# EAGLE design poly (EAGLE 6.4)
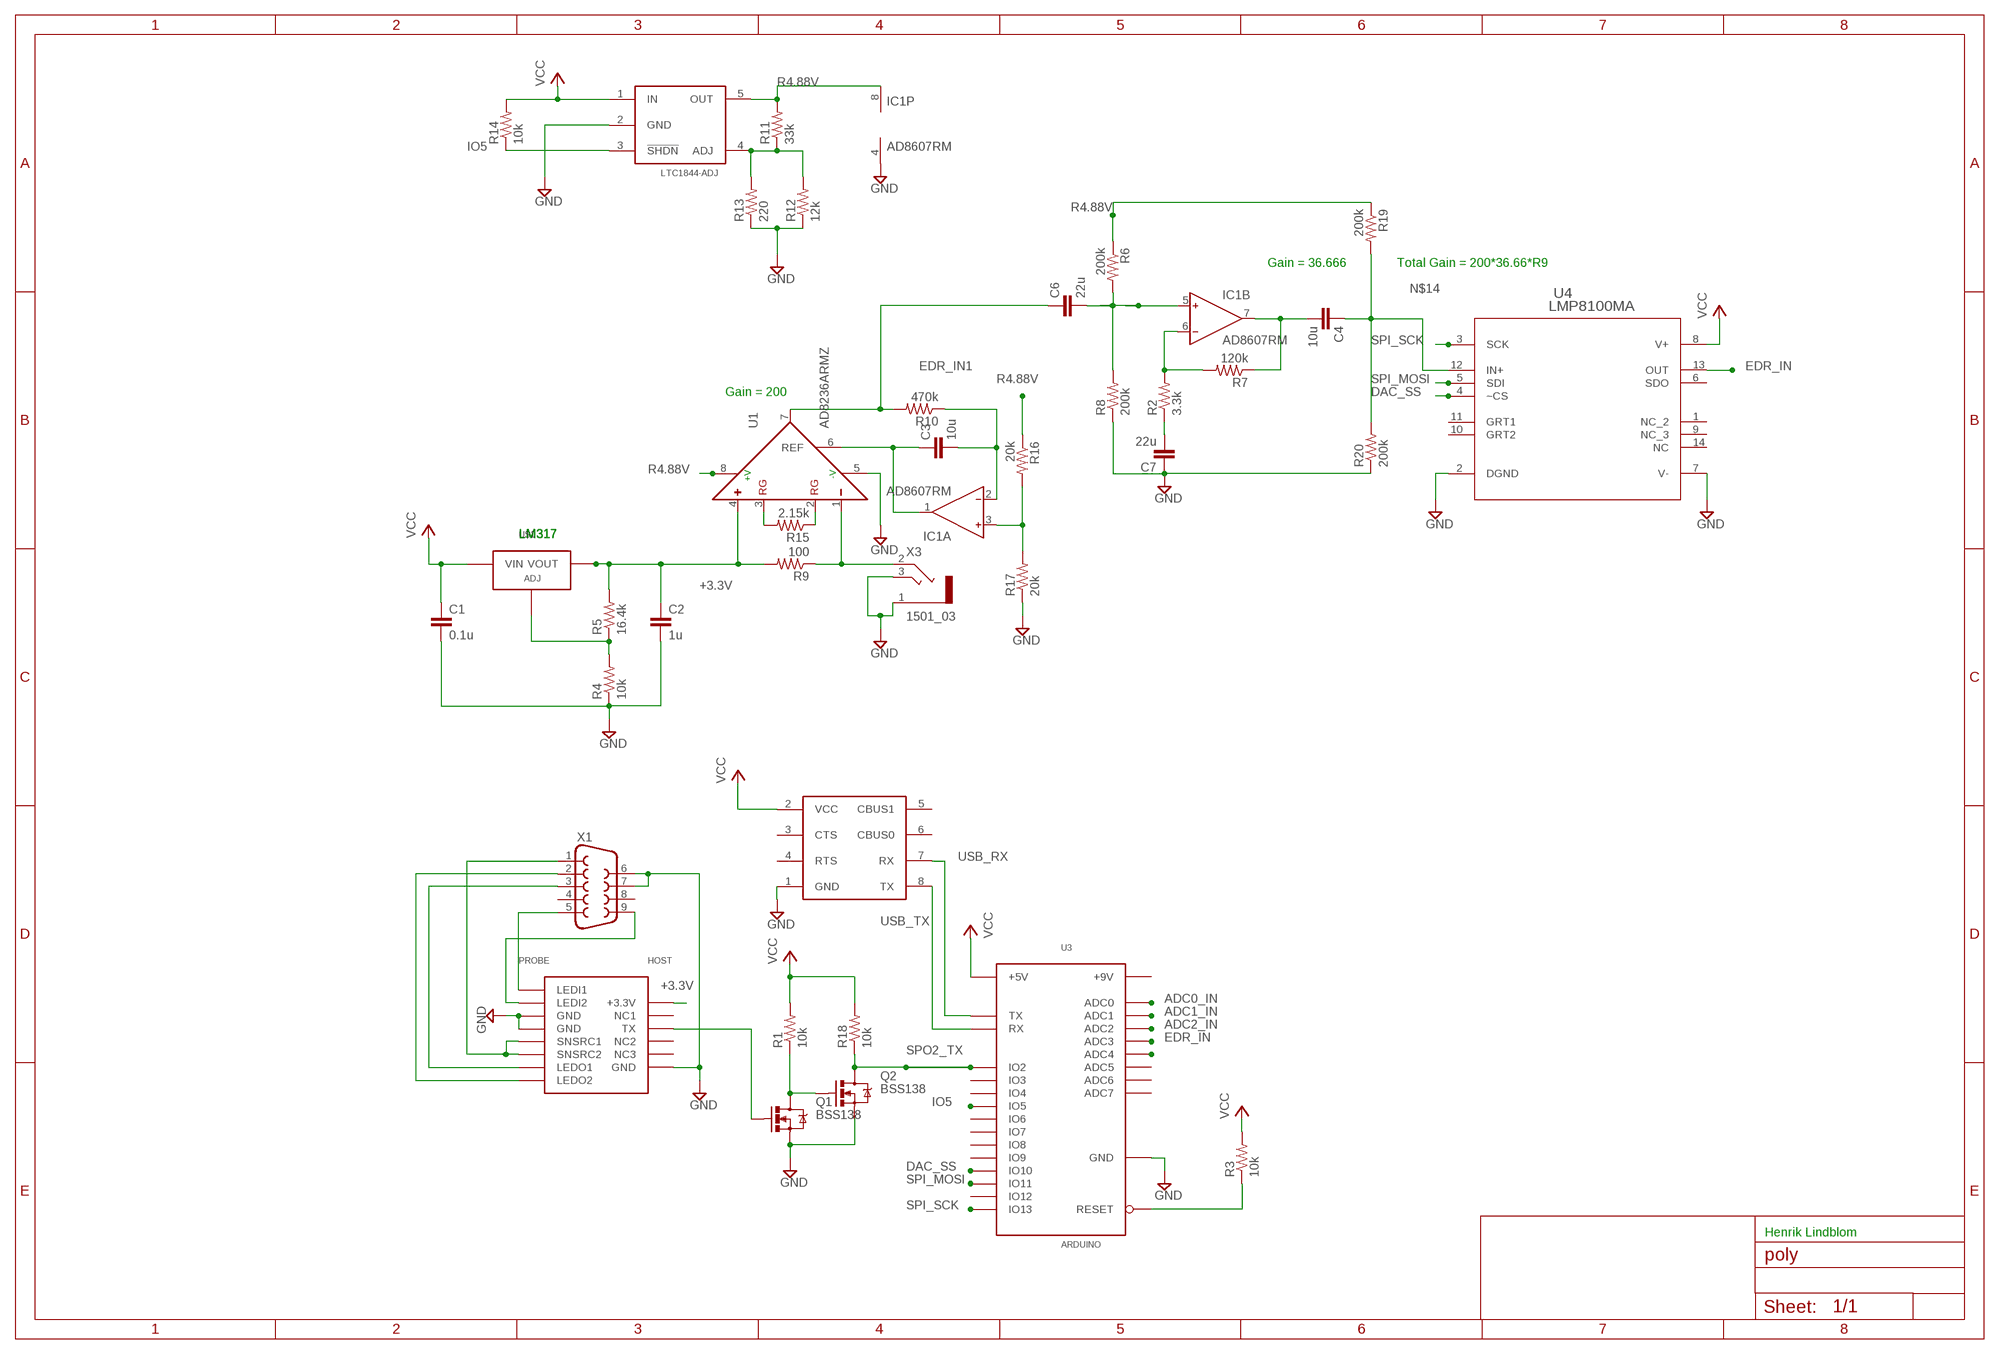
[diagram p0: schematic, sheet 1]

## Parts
C1  0.1u  C-EUC0603K  [C0603K]
C2  1u  C-EUC0805K  [C0805K]
C3  10u  C-EUC0805K  [C0805K]
C4  10u  C-EUC0603  [C0603]
C6  22u  C-EUC0805K  [C0805K]
C7  22u  C-EUC0805K  [C0805K]
IC1  AD8607RM  [MSOP08]
MEDLABSPO2  MEDLAB_SPO2  [MEDLAB_SPO2]
Q1  BSS138  BSS138TRANS-00830  [SOT23-3]
Q2  BSS138  BSS138TRANS-00830  [SOT23-3]
R1  10k  RESISTOR0805-RES  [0805]
R2  3.3k  RESISTOR0805-RES  [0805]
R3  10k  RESISTOR0805-RES  [0805]
R4  10k  RESISTOR0805-RES  [0805]
R5  16.4k  RESISTOR0805-RES  [0805]
R6  200k  RESISTOR0805-RES  [0805]
R7  120k  RESISTOR0805-RES  [0805]
R8  200k  RESISTOR0805-RES  [0805]
R9  100  RESISTOR0805-RES  [0805]
R10  470k  RESISTOR0805-RES  [0805]
R11  33k  RESISTOR0805-RES  [0805]
R12  12k  RESISTOR0805-RES  [0805]
R13  220  RESISTOR0805-RES  [0805]
R14  10k  RESISTOR0805-RES  [0805]
R15  2.15k  RESISTOR0805-RES  [0805]
R16  20k  RESISTOR0603-RES  [0603-RES]
R17  20k  RESISTOR0603-RES  [0603-RES]
R18  10k  RESISTOR0805-RES  [0805]
R19  200k  RESISTOR0603-RES  [0603-RES]
R20  200k  RESISTOR0603-RES  [0603-RES]
U1  AD8236ARMZ  [SOP65P490X110-8N]
U2  UB232R  [UB232R]
U3  ARDUINO  [ARDUINO_MINI]
U4  LMP8100MA  [M14A]
U$1  LM317  [SOT-89]
U$5  LTC1844-ADJ  [SOT23-5]
X1  F09HP  [F09HP]
X3  1501_03  [1501_03]

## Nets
+3.3V: C2.1 MEDLABSPO2.+3.3V R5.2 R9.2 U1.4(+) U$1.P$1(VOUT) U$1.P$2(VOUT)
ADC0_IN: U3.ADC0
ADC1_IN: U3.ADC1
ADC2_IN: U3.ADC2
ADC4_IN: U3.ADC4
DAC_SS: U3.IO10 U4.4(~CS)
EDR_IN: U3.ADC3 U4.13(OUT)
EDR_IN1: C3.2 IC1.2(A:IN-) R10.1
EDR_IN2: C4.2 IC1.7(B:OUT) R7.1
GND: C1.2 C2.2 C7.1 IC1.4(P:V-) MEDLABSPO2.GND MEDLABSPO2.GND@1(GND) MEDLABSPO2.GND@2(GND) Q1.2(S) Q2.2(S) R4.1 R8.1 R12.1 R13.1 R17.1 R20.1 U1.5(-V) U2.1(GND) U3.GND U4.2(DGND) U4.7(V-) U$5.2(GND) X1.6 X1.7 X3.1 X3.3
IO5: R14.1 U3.IO5 U$5.3(!SHDN)
N$1: MEDLABSPO2.LEDI1 X1.5
N$2: MEDLABSPO2.LEDI2 X1.9
N$3: MEDLABSPO2.SNSRC1 MEDLABSPO2.SNSRC2 X1.1
N$4: MEDLABSPO2.LEDO1 X1.3
N$5: MEDLABSPO2.LEDO2 X1.2
N$6: R3.1 U3.RESET
N$9: MEDLABSPO2.TX Q1.1(G)
N$10: Q1.3(D) Q2.1(G) R1.1
N$11: R4.2 R5.1 U$1.P$3(ADJ)
N$12: IC1.6(B:IN-) R2.2 R7.2
N$13: C6.1 R10.2 U1.7(OUT)
N$14: C4.1 R19.2 R20.2 U4.12(IN+)
N$15: IC1.3(A:IN+) R16.2 R17.2
N$17: C7.2 R2.1
N$18: C3.1 IC1.1(A:OUT) U1.6(REF)
N$20: R9.1 U1.1(-) X3.2
N$21: R11.1 R12.2 R13.2 U$5.4(ADJ)
N$22: C6.2 IC1.5(B:IN+) R6.2 R8.2
N$23: R15.2 U1.3(RG)
N$24: R15.1 U1.2(RG)
R4.88V: IC1.8(P:V+) R6.1 R11.2 R16.1 R19.1 U1.8(+V) U$5.5(OUT)
SPI_MOSI: U3.IO11 U4.5(SDI)
SPI_SCK: U3.IO13 U4.3(SCK)
SPO2_TX: Q2.3(D) R18.1 U3.IO2
USB_RX: U2.7(RX) U3.TX
USB_TX: U2.8(TX) U3.RX
VCC: C1.1 R1.2 R3.2 R14.2 R18.2 U2.2(VCC) U3.+5V U4.8(V+) U$1.P$4(VIN) U$5.1(IN)
Unconnected: MEDLABSPO2.NC@1(NC1) MEDLABSPO2.NC@2(NC2) MEDLABSPO2.NC@3(NC3) U2.3(CTS) U2.4(RTS) U2.5(CBUS1) U2.6(CBUS0) U3.ADC5 U3.ADC6 U3.ADC7 U3.IO3 U3.IO4 U3.IO6 U3.IO7 U3.IO7@1(IO7) U3.IO8 U3.IO9 U3.IO12 U3.RESET@1(RESET) U3.RX@1(RX) U3.TX@1(TX) U4.1(NC_2) U4.6(SDO) U4.9(NC_3) U4.10(GRT2) U4.11(GRT1) U4.14(NC) X1.4 X1.8

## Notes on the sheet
- Gain = 36.666 | Total Gain = 200*36.66*R9
- Gain = 200
- LM317 | LM317 | LM317
- Henrik Lindblom

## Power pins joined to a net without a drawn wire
+5V: U3.+5V@2(+5V) U3.P$31(+5V)
+9V: U3.+9V
GND: U3.GND@2(GND) U3.GND@3(GND) U3.GND@4(GND)

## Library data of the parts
C1-C4 C6 C7 = rcl:C-EU: CAPACITOR, European symbol
IC1 = analog-devices:AD8607: Precision Micropower, Low Noise CMOS, Rail-to-Rail Input/Output Operational Amplifiers Source: http://www.analog.com/static/imported-files/data_sheets/AD8603_8607_8609.pdf; MF: ALTERA CORPORATION; MPN: AD8607ARMZ-REEL; OC_FARNELL: 1464990; OC_NEWARK: 59K6925
MEDLABSPO2 = poly:MEDLAB_SPO2
Q1 Q2 = SparkFun-DiscreteSemi:BSS138: NMOSFET, Enh Mode 50V/6-ohm 200mA (SOT-23) TRANS-00830; PROD_ID: TRANS-00830
R1 R3 R18 = SparkFun-Resistors:RESISTOR: Resistor
R2 R4-R17 R19 R20 = SparkFun-Resistors:RESISTOR: Resistor; TOLERANCE: 1%
U1 = Analog Devices_By_element14_Batch_1:AD8236ARMZ: 40 uA Micropower Instrumentation Amplifier with Zero Crossover Distortion; MPN: AD8236ARMZ; OC_FARNELL: 1827362; OC_NEWARK: 80R8173; PACKAGE: MSOP-8; SUPPLIER: Analog Devices
U2 = poly:UB232R
U3 = poly:ARDUINO
U4 = ti_lmp8100:LMP8100MA
U$1 = poly:LM317
U$5 = poly:LTC1844-ADJ
X1 = con-subd:F09: SUB-D; OC_FARNELL: unknown; OC_NEWARK: unknown
X3 = con-lumberg:1501_03: Klinkensteckverbinder nach JISC 6560, 2,5 mm Jack connectors according to JISC 6560, 2.5 mm Source: http://www.lumberg.com/Produkte/PDFs/1501_03.pdf; OC_FARNELL: 1200127; OC_NEWARK: unknown

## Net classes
0 default: clearance 0.025 mm

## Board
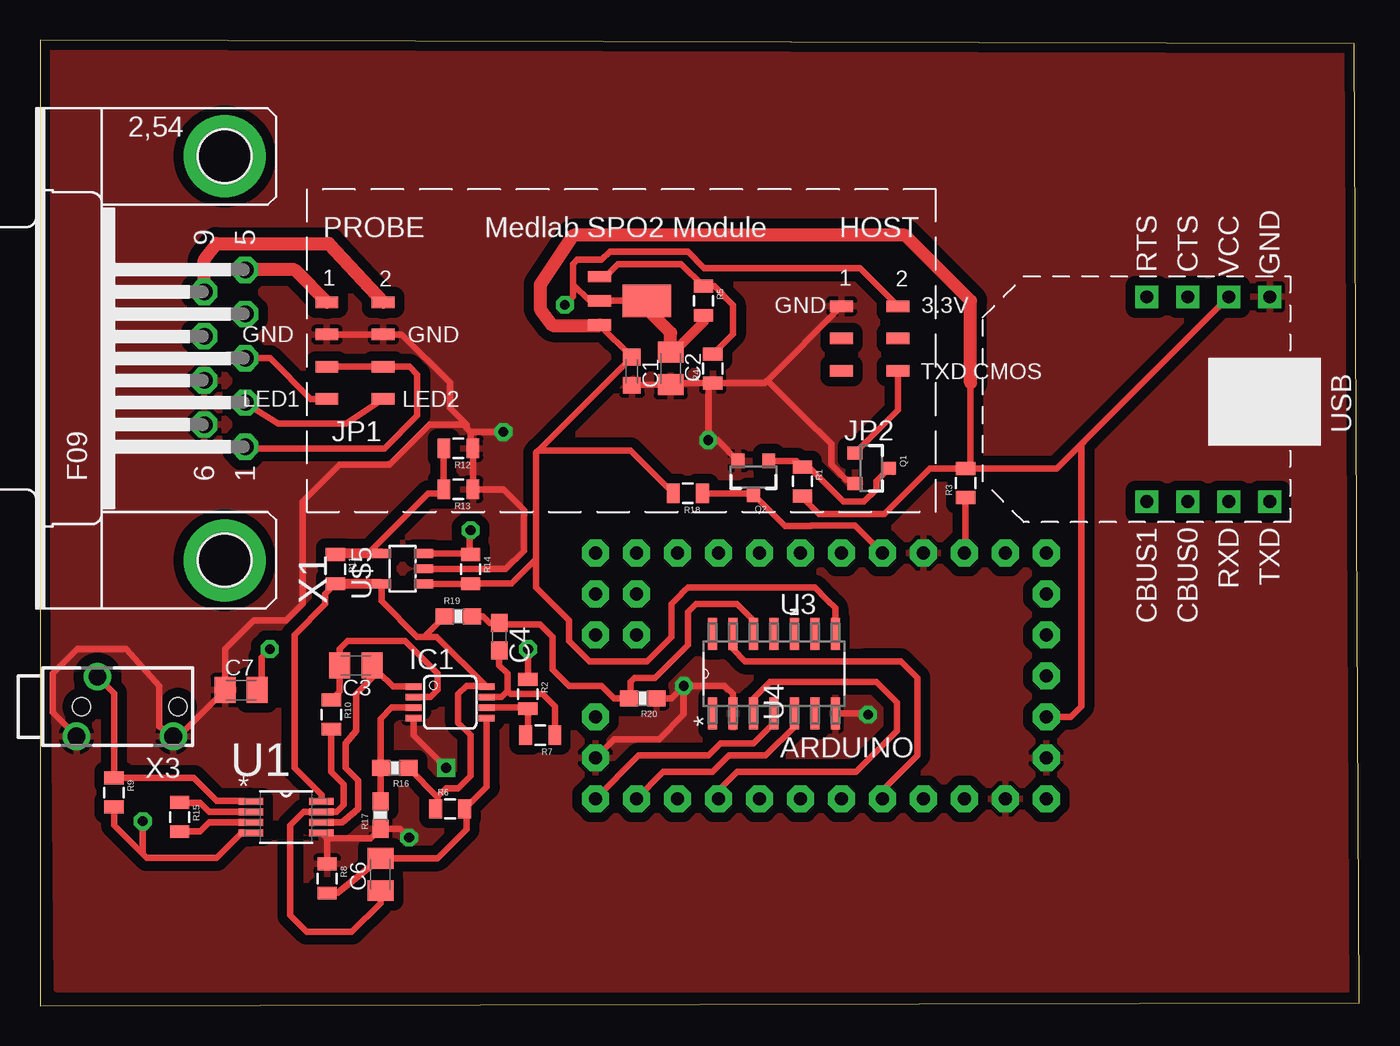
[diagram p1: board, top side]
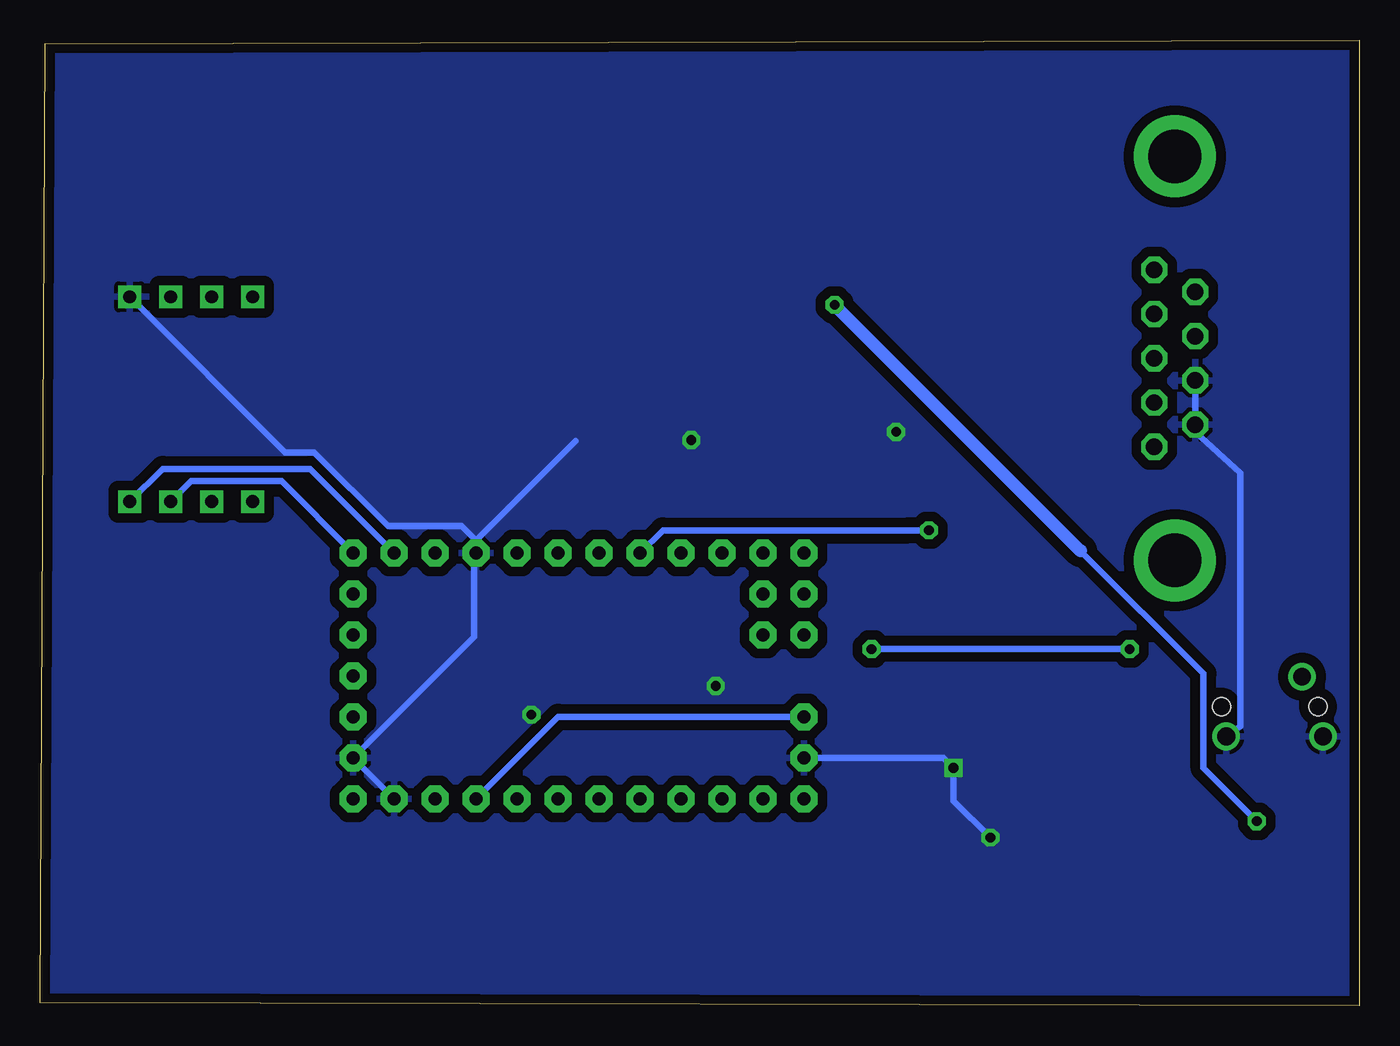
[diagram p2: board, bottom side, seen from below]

Size 81.74 x 59.83 mm. Coordinates in mm from the lower left corner, seen from the top.
Outline: 0,0 81.74,0.16 81.44,59.62 0,59.83 0,0
Copper layers (1*16): Top 0.035mm / dielectric 1.5mm / Bottom 0.035mm
Design rules "SparkFun": minimum track width 8mil, minimum drill 20mil, track to track 8mil, track to pad 8mil, pad to pad 8mil, via to via 8mil, smd to smd 8mil, copper to edge 10mil, drill to drill 8mil, minimum pad ring 12mil, minimum via ring 10mil, stop-mask expansion 4mil, vias tented up to drill 25mil, thermal gap 10mil

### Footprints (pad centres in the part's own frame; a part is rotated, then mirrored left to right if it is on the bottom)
C0603K = smd 1.05 x 1.08: 1 -0.875,0; 2 0.875,0
C0805K = smd 1.3 x 1.6: 1 -1,0; 2 1,0
C0603 = smd 1.1 x 1: 1 -0.85,0; 2 0.85,0
MSOP08 = smd 0.4 x 1: 1 -0.976,-2.263; 2 -0.326,-2.263; 3 0.324,-2.263; 4 0.974,-2.263; 5 0.974,2.262; 6 0.324,2.262; 7 -0.326,2.262; 8 -0.976,2.262
MEDLAB_SPO2 = smd 1.422 x 0.711: +3.3V 33.65,2.75; GND 30.15,2.75; GND@1 -1.75,1; GND@2 1.75,1; LEDI1 -1.75,3; LEDI2 1.75,3; LEDO1 -1.75,-3; LEDO2 1.75,-3; NC@1 30.15,0.75; NC@2 33.65,0.75; NC@3 30.15,-1.25; SNSRC1 -1.75,-1; SNSRC2 1.75,-1; TX 33.65,-1.25
SOT23-3 = smd 0.8 x 0.9: 1 -0.95,-1; 2 0.95,-1; 3 0,1.1
0805 = smd 0.8 x 1.2: 1 -0.9,0; 2 0.9,0
0603-RES = smd 1.1 x 1: 1 -0.85,0; 2 0.85,0
SOP65P490X110-8N = smd 1.499 x 0.432: 1 -2.184,0.965; 2 -2.184,0.33; 3 -2.184,-0.33; 4 -2.184,-0.965; 5 2.184,-0.965; 6 2.184,-0.33; 7 2.184,0.33; 8 2.184,0.965
UB232R = drill 0.8 square: 1 -7.62,-6.35; 2 -5.08,-6.35; 3 -2.54,-6.35; 4 0,-6.35; 5 0,6.35; 6 -2.54,6.35; 7 -5.08,6.35; 8 -7.62,6.35
ARDUINO_MINI = drill 0.8 pad 1.676 octagon: +5V 11.43,29.21; +5V@2 16.51,21.59; +9V 16.51,29.21; ADC0 16.51,11.43; ADC1 16.51,13.97; ADC2 16.51,16.51; ADC3 16.51,19.05; ADC4 3.81,1.27; ADC5 6.35,1.27; ADC6 3.81,3.81; ADC7 6.35,3.81; GND 13.97,29.21; GND@2 16.51,26.67; GND@3 1.27,21.59; GND@4 13.97,1.27; IO2 1.27,19.05; IO3 1.27,16.51; IO4 1.27,13.97; IO5 1.27,11.43; IO6 1.27,8.89; IO7 1.27,6.35; IO7@1 3.81,29.21; IO8 1.27,3.81; IO9 1.27,1.27; IO10 16.51,1.27; IO11 16.51,3.81; IO12 16.51,6.35; IO13 16.51,8.89; P$31 11.43,1.27; RESET 1.27,24.13; RESET@1 16.51,24.13; RX 1.27,26.67; RX@1 8.89,29.21; TX 1.27,29.21; TX@1 6.35,29.21
M14A = smd 1.981 x 0.559: 1 -2.464,3.81; 2 -2.464,2.54; 3 -2.464,1.27; 4 -2.464,0; 5 -2.464,-1.27; 6 -2.464,-2.54; 7 -2.464,-3.81; 8 2.464,-3.81; 9 2.464,-2.54; 10 2.464,-1.27; 11 2.464,0; 12 2.464,1.27; 13 2.464,2.54; 14 2.464,3.81
SOT-89 = smd 2 x 3: P$1 0,1.778 | smd 0.711 x 1.422: P$2 0,-1.143; P$3 -1.499,-1.143; P$4 1.499,-1.143
SOT23-5 = smd 0.55 x 1.2: 1 -1.05,-1.4; 2 -0.1,-1.4; 3 0.85,-1.4; 4 0.85,1.2; 5 -1.05,1.2
F09HP = drill 1.016 octagon: 1 -5.486,-1.27; 2 -2.743,-1.27; 3 0,-1.27; 4 2.743,-1.27; 5 5.486,-1.27; 6 -4.115,1.27; 7 -1.372,1.27; 8 1.372,1.27; 9 4.115,1.27 | drill 3.302 pad 5.08: G1 -12.522,0; G2 12.522,0
1501_03 = drill 1.1 pad 1.7: 1 -1.85,0.3; 2 1.85,-1; 3 -1.85,-5.7 | hole 1.1: 0,0; 0,-6

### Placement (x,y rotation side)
C1  36.66,39.32 270 top
C2  39.07,39.49 270 top
C3  19.56,21.08 180 top
C4  28.45,22.86 270 top
C6  21.08,8.13 90 top
C7  12.45,19.56 0 top
IC1  25.4,18.8 270 top
MEDLABSPO2  19.51,40.6 0 top
Q1  51.49,33.3 270 top
Q2  44.2,32.77 180 top
R1  47.24,32.49 270 top
R2  30.23,19.3 270 top
R3  57.35,32.39 90 top
R4  41.68,39.48 90 top
R5  41.11,43.69 270 top
R6  25.4,12.19 0 top
R7  30.99,16.76 180 top
R8  17.78,7.87 270 top
R9  4.57,13.21 270 top
R10  18.03,18.03 270 top
R11  18.29,27.05 270 top
R12  25.91,34.54 180 top
R13  25.91,32 180 top
R14  26.67,27.05 270 top
R15  8.64,11.68 270 top
R16  21.97,14.73 180 top
R17  21.08,11.81 90 top
R18  40.13,31.75 180 top
R19  25.91,24.13 0 top
R20  37.34,19.05 180 top
U1  15.24,11.68 0 top
U2  68.58,37.58 180 top
U3  33.14,29.32 270 top
U4  45.47,20.57 90 top
U$1  35.81,43.69 270 top
U$5  22.35,27.18 90 top
X1  11.43,40.12 90 top
X3  2.54,18.53 90 top

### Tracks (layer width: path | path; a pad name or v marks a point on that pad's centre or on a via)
+3.3V  (via drill 0.6)
  Top 0.406: R5.2 41.11,42.53 41.11,42.38 | 37.6,43.69 U$1.P$1 37.08,43.69 U$1.P$2 34.04,43.69 33.02,44.7 | 33.02,44.7 33.02,45.97 33.27,46.23 34.8,46.23 35.31,46.74 40.13,46.74 41.15,45.72 50.79,45.72 MEDLABSPO2.+3.3V | 39.62,40.89 39.47,40.89 C2.1 | R9.2 4.57,11.18 6.35,9.4 | 6.35,9.4 6.6,9.14 10.92,9.14 12.45,10.67 13.01,10.67 U1.4 12.5,10.72 | 33.02,44.7 33.02,43.94 v32.51,43.43 | v6.35,11.43 6.35,9.4
  Top 0.61: 41.11,42.38 39.62,40.89
  Top 0.813: C2.1 39.07,41.7 37.08,43.69
  Bottom 0.406: v6.35,11.43 9.65,14.73 9.65,20.57 17.27,28.19
  Bottom 0.813: 17.27,28.19 v32.51,43.43
+5V
  Bottom 0.406: U3.+5V@2 49.65,17.89 U3.P$31
DAC_SS
  Top 0.406: U3.IO10 37.08,15.49 41.4,15.49 42.16,16.26 44.2,16.26 45.47,17.53 U4.4
EDR_IN
  Top 0.406: U4.13 42.93,22.1 43.69,21.34 51.05,21.34 53.34,21.34 54.36,20.32 54.36,15.49 52.19,13.33 U3.ADC3
EDR_IN1
  Top 0.406: R10.1 18.56,19.46 C3.2 18.54,21.1 18.54,22.1 19.05,22.61 22.61,22.61 23.11,22.1 24.64,20.57 24.64,19.56 24.2,19.12 IC1.2
EDR_IN2
  Top 0.406: IC1.7 28.57,19.13 28.96,19.51 | 28.96,19.51 28.96,20.57 28.45,21.08 C4.2 | 28.96,19.51 29.13,19.33 31.11,19.33 31.89,18.56 R7.1
GND  (via drill 0.6)
  Top 0.406: 39.16,38.58 C2.2 | R4.1 44.89,38.58 45.06,38.76 | 45.06,38.76 MEDLABSPO2.GND | R4.1 39.16,38.58 | 39.16,38.58 C2.2 | C1.2 38.46,38.49 C2.2 | MEDLABSPO2.GND@1 MEDLABSPO2.GND@2 22.4,41.6 25.4,38.61 25.4,37.02 26.42,36.01 26.42,35.81 26.67,35.56 | U$5.2 23.78,27.05 28.83,27.05 29.97,28.19 29.97,30.73 28.7,32 R13.1 R12.1 26.67,34.68 26.67,35.56 | R8.1 17.78,10.36 | 17.78,10.36 U1.5 | 26.67,35.56 26.22,36.01 24.13,36.01 21.65,33.53 18.54,33.53 16.26,31.24 16.26,24.89 15.24,23.88 13.21,23.88 11.45,22.11 C7.1 8.57,16.68 X3.3 7.37,17.3 7.37,19.81 5.33,22.1 2.29,22.1 0.76,20.57 0.76,19.05 0.76,18.16 X3.1 | 45.06,38.76 47.24,36.58 49.02,34.8 49.02,33.53 49.94,32.61 Q1.2 | IC1.4 23.14,16.74 v25.15,14.73 | v22.86,10.41 22.31,10.96 R17.1 20.48,10.36 17.78,10.36 | 26.67,35.56 v28.7,35.56 | U4.7 51.23,18.11 v51.31,18.03 | U4.2 42.93,19.3 42.42,19.81 v39.88,19.81 | R4.1 41.4,38.31 v41.4,35.05 41.96,35.05 Q2.2 | U3.GND@4 35.57,16.51 38.35,16.51 39.88,18.03 v39.88,19.81 | v39.88,19.81 39.12,19.05 R20.1
  Bottom 0.406: U2.1 66.56,34.29 64.77,34.29 60.2,29.72 55.63,29.72 54.73,28.82 | 54.73,28.82 U3.GND@3 54.73,27.57 54.86,27.43 54.86,22.84 U3.GND U3.GND@2 | 54.73,28.82 48.56,34.99 | X1.7 X1.6 10.16,35.56 7.37,33.02 7.37,17.3 X3.3 | U3.GND@4 25.77,15.35 v25.15,14.73 25.15,12.7 v22.86,10.41
  pour Bottom (isolate 0.61): 0.25,0.25 0.25,59.44 81.53,59.44 81.53,0.51 0.51,0.51
  pour Top (isolate 0.61): 0.51,59.44 81.28,59.44 81.03,1.02 1.02,1.02
IO5  (via drill 0.6)
  Top 0.406: R14.1 26.59,28.03 | 26.59,28.03 U$5.3 | 26.59,28.03 26.59,29.39 v26.67,29.46
  Bottom 0.406: U3.IO5 43.16,29.46 27.94,29.46 v26.67,29.46
N$1
  Top 0.61: 17.86,43.6 MEDLABSPO2.LEDI1
  Top 0.813: MEDLABSPO2.LEDI1 15.75,45.61 X1.5
N$2
  Top 0.813: X1.9 10.16,46.23 10.92,47.24 17.87,47.24 MEDLABSPO2.LEDI2
N$3
  Top 0.406: X1.1 12.79,34.54 21.34,34.54 23.37,36.58 23.37,39.12 22.88,39.6 MEDLABSPO2.SNSRC2 MEDLABSPO2.SNSRC1
N$4
  Top 0.406: X1.3 14.23,40.12 16.76,37.59 17.75,37.59 MEDLABSPO2.LEDO1
N$5
  Top 0.406: X1.2 12.7,37.34 14.73,36.07 18.96,36.07 MEDLABSPO2.LEDO2
N$6
  Top 0.406: R3.1 57.35,28.13 U3.RESET
N$9
  Top 0.406: Q1.1 53.16,36.92 MEDLABSPO2.TX
N$10
  Top 0.406: 52.83,33.06 Q1.3 51.82,32.53 51.82,32 51.05,31.24 50.55,31.24 50.04,31.24 49.78,31.24 47.63,33.39 R1.1 46.87,33.77 Q2.1
N$11
  Top 0.406: U$1.P$3 35.03,45.19 35.81,45.97 39.72,45.97 R5.1 41.77,44.59 42.93,43.43 42.93,41.63 R4.2
N$12
  Top 0.406: R7.2 30.23,16.9 R2.2 30.16,18.47 IC1.6
N$13
  Top 0.406: C6.1 21.08,6.35 19.3,4.57 16.51,4.57 15.49,5.59 15.49,11.18 16.33,12.01 U1.7 18.36,12.01 18.8,12.45 18.8,13.72 18.03,14.48 R10.2
N$14
  Top 0.406: R19.2 27.43,24.13 27.85,23.71 C4.1 28.54,23.62 30.48,23.62 30.99,23.62 31.75,22.86 31.75,20.83 32.77,19.81 34.8,19.81 35.56,19.05 R20.2 36.58,19.14 36.58,20.07 36.83,20.32 37.59,20.32 38.1,20.32 40.13,22.35 40.13,24.38 40.64,24.89 43.18,24.89 44.2,23.88 U4.12
N$15
  Top 0.406: R17.2 21.08,14.69 R16.2 21.08,14.77 21.08,17.78 21.77,18.47 IC1.3
N$17  (via drill 0.6)
  Top 0.406: C7.2 13.72,19.83 13.72,21.59 v14.22,22.1 | R2.1 v30.23,22.1
  Bottom 0.406: v14.22,22.1 v30.23,22.1
N$18
  Top 0.406: IC1.1 21.87,19.77 20.95,20.69 | 20.95,20.69 C3.1 | U1.6 18.72,11.35 19.68,12.19 19.68,13.97 18.92,14.73 18.92,16.26 19.56,17.02 19.56,19.3 19.81,19.56 20.95,20.69
N$20
  Top 0.406: U1.1 13.01,12.7 10.92,12.7 9.51,14.11 R9.1 4.57,19.35 X3.2
N$21
  Top 0.406: 18.34,28.03 R11.1 | R12.2 R13.2 25.15,31.87 25.15,31.75 24.04,31.75 20.32,28.03
  Top 0.61: U$5.4 20.32,28.03 18.34,28.03
N$22
  Top 0.406: IC1.5 27.66,13.55 R6.2 26.42,12.08 26.42,10.92 24.62,9.13 C6.2 18.42,6.97 R8.2
N$23
  Top 0.406: U1.3 10.46,11.35 9.91,10.79 8.65,10.79 R15.2
N$24
  Top 0.406: U1.2 10.46,12.01 9.91,12.57 R15.1
R4.88V
  Top 0.406: 18.44,26.13 R11.2 17.65,25.52 17.65,24.89 15.75,22.99 15.75,14.73 16.26,14.22 17.42,13.06 U1.8 | U$5.5 21.15,25.08 23.37,22.86 23.62,22.86 | 23.62,22.86 24.57,22.86 IC1.8 27.62,19.81 26.42,19.81 25.91,19.3 25.91,17.53 26.67,16.76 26.67,14.22 25.91,13.46 25.15,13.46 24.64,12.95 24.64,12.7 | 24.64,12.7 24.64,12.19 R6.1 | R16.1 24.64,12.91 24.64,12.7 | R19.1 23.79,22.86 23.62,22.86
  Top 0.61: U$5.5 18.44,26.13
SPI_MOSI
  Top 0.406: 36.83,12.7 36.84,12.7 U3.IO11 38.61,14.48 41.66,14.48 42.67,15.49 44.96,15.49 46.74,17.27 U4.5
SPI_SCK
  Top 0.406: U3.IO13 42.03,13.33 43.18,14.48 50.55,14.48 53.09,17.02 53.09,18.8 51.82,20.07 45.21,20.07 44.2,19.05 U4.3
SPO2_TX
  Top 0.406: U3.IO2 50.49,29.75 47.79,29.75 47.75,29.72 46.14,29.72 Q2.3 44.11,31.75 R18.1
USB_RX
  Bottom 0.406: U2.7 72.38,32.51 66.8,32.51 U3.TX
USB_TX
  Bottom 0.406: U2.8 74.16,33.27 65.02,33.27 U3.RX
VCC
  Top 0.406: R3.2 57.34,33.3 57.66,33.63 57.66,38.86 | 30.87,34.41 C1.1 U$1.P$4 | 30.87,34.41 30.73,34.27 30.73,27.69 | 30.73,27.69 29.2,26.15 R14.2 26.65,26.13 U$5.1 | U2.2 64.9,35.17 | 64.9,35.17 64.52,34.79 64.52,18.54 63.87,17.89 U3.+5V | R3.2 63.02,33.29 64.9,35.17 | 30.73,27.69 30.73,25.91 32.77,23.88 32.77,22.61 34.04,21.34 34.8,21.34 37.59,21.34 38.86,22.61 39.12,22.86 39.12,24.89 39.62,25.4 39.88,25.65 40.13,25.91 48.01,25.91 48.77,25.15 49.28,24.64 U4.8 | R18.2 36.58,34.41 30.87,34.41 | R1.2 47.24,31.5 48.26,30.48 52.32,30.48 55.13,33.29 R3.2
  Top 0.813: 57.66,38.61 57.66,38.86 57.66,43.69 53.59,47.75 33.02,47.75 30.99,44.7 30.99,43.18 31.75,42.16 34.65,42.16 U$1.P$4

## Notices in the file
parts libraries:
SparkFun-DiscreteSemi: Licensing: CC v3.0 Share-Alike You are welcome to use this library for commercial purposes.
